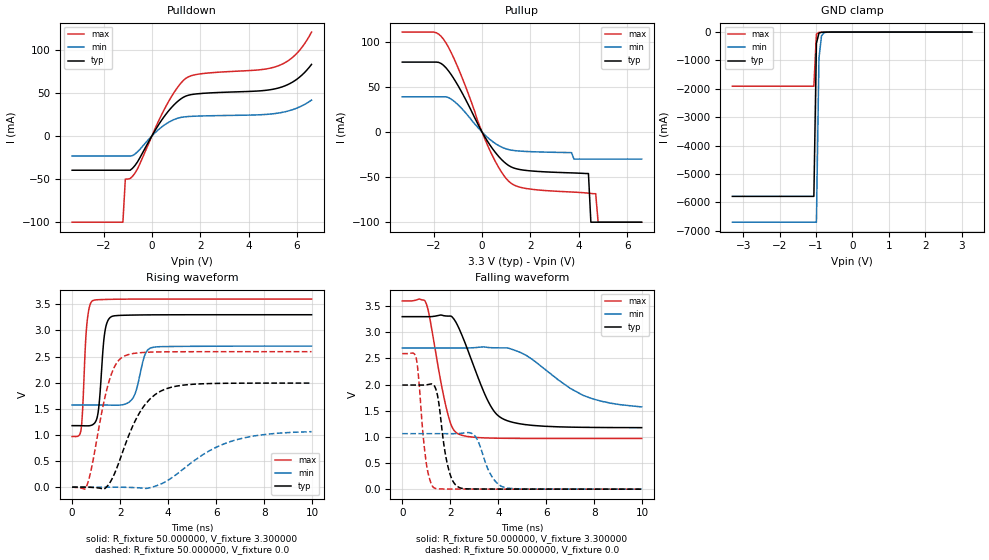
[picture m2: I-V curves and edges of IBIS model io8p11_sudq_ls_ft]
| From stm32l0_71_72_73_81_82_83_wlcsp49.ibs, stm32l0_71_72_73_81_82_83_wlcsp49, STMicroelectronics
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|   Model io8p11_sudq_ls_ft
[Model]  io8p11_sudq_ls_ft
Model_type I/O
Polarity   Non-Inverting
Enable   Active-Low
Vinl =   0.990000V
Vinh =   2.310000V
Vmeas =  1.650000V
Cref =   50.000000pF
Rref =   100.000000M
Vref =   0.0V
C_comp   2.343000pF   2.309800pF   2.393900pF
[Temperature Range]   25.000000   0.125000k   -40.000000
[Pullup Reference]   3.300000V   2.700000V   3.600000V
[Pulldown Reference]   0.0V   0.0V   0.0V
[POWER Clamp Reference]   3.300000V   2.700000V   3.600000V
[GND Clamp Reference]   0.0V   0.0V   0.0V
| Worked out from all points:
|   slope of the pulldown table from 0 to 0.495 V, typ, clamps not added: 22.6 ohm
|   slope of the pullup table from 0 to 0.495 V, typ, clamps not added: 23.9 ohm
|   GND clamp passes 1 mA (typ) near -0.64 V on its own axis
|   rising waveform, R_fixture 50.000000, V_fixture 3.300000: 20-80 % time 209ps typ, 360ps min, 167ps max; typ from 1.18 V to 3.3 V
|   rising waveform, R_fixture 50.000000, V_fixture 0.0: 20-80 % time 1.18ns typ, 2.2ns min, 697ps max; typ from 0 V to 1.99 V
|   falling waveform, R_fixture 50.000000, V_fixture 3.300000: 20-80 % time 1.12ns typ, 2.08ns min, 643ps max; typ from 3.3 V to 1.18 V
|   falling waveform, R_fixture 50.000000, V_fixture 0.0: 20-80 % time 383ps typ, 558ps min, 304ps max; typ from 1.99 V to 0 V
[Pulldown]
|Voltage   I(typ)   I(min)   I(max)
-3.3V     -39.8mA    -23.37mA   -100mA
-1.2V     -39.8mA    -23.37mA   -100mA
-1.1V     -39.8mA    -23.37mA   -50.1mA
-900mV    -39.8mA    -23.37mA   -49.43mA
-700mV    -34.25mA   -21mA      -43.13mA
600mV     25.84mA    14.18mA    35.34mA
1V        38.32mA    19.82mA    53.81mA
1.4V      46.09mA    22.19mA    66.63mA
2V        49.05mA    23.02mA    71.83mA
5.2V      55.23mA    26.32mA    80.92mA
6V        65.76mA    32.26mA    95.84mA
6.6V      82.81mA    41.43mA    120.2mA
[Pullup]
|Voltage   I(typ)   I(min)   I(max)
-3.3V     77.63mA    39.16mA    110.9mA
-2V       77.63mA    39.16mA    110.9mA
-1.6V     74.23mA    39.16mA    103.2mA
-900mV    47.13mA    27.82mA    65.37mA
300mV     -13.29mA   -7.65mA    -18.99mA
1.2V      -38.62mA   -20mA      -56.79mA
3.7V      -45.29mA   -22.8mA    -66.5mA
4.4V      -46mA      -30mA      -67.77mA
4.5V      -100mA     -30mA      -68.06mA
4.7V      -100mA     -30mA      -68.4mA
4.8V      -100mA     -30mA      -100mA
6.6V      -100mA     -30mA      -100mA
[GND_clamp]
|Voltage   I(typ)   I(min)   I(max)
-3.3V     -5.787A    -6.696A    -1.906A
-1.06V    -5.787A    -6.696A    -1.906A
-990mV    -393.4mA   -6.696A    -70.75mA
-920mV    -33.02mA   -919.4mA   -10.9mA
-850mV    -6.829mA   -131.3mA   -6.521mA
-780mV    -3.478mA   -21.06mA   -4.208mA
3.28V     0A         0A         0A
[POWER_clamp]
|Voltage   I(typ)   I(min)   I(max)
-3.28V    0A         0A         0A
0V        0A         0A         0A
[Ramp]
| variable   typ   min   max
dV/dt_r  1.19466/1.17578n   0.61164/2.08555n   1.55562/0.69590n
dV/dt_f  1.27212/1.11937n   0.59256/1.87709n   1.57784/0.64179n
R_load = 50.000000
[Rising Waveform]
R_fixture= 50.000000
V_fixture= 3.300000
V_fixture_min= 2.700000
V_fixture_max= 3.600000
|time   V(typ)   V(min)   V(max)
0s        1.177V     1.573V     969.2mV
380.4ps   1.176V     1.573V     1.129V
600.6ps   1.173V     1.573V     3.051V
860.9ps   1.196V     1.573V     3.57V
1.101ns   1.494V     1.573V     3.588V
1.381ns   3.02V      1.572V     3.592V
1.642ns   3.264V     1.569V     3.595V
2.523ns   3.294V     1.699V     3.599V
3.283ns   3.298V     2.666V     3.6V
9.97ns    3.3V       2.7V       3.6V
[Rising Waveform]
R_fixture= 50.000000
V_fixture= 0.0
V_fixture_min= 0.0
V_fixture_max= 0.0
|time   V(typ)   V(min)   V(max)
0s        -3.21uV    7.798uV    -231.3uV
620.6ps   -747.1uV   -8.107uV   39.58mV
820.8ps   -5.23mV    3.783uV    394.6mV
1.502ns   39.32mV    181.5uV    1.968V
1.802ns   299.1mV    -186.8uV   2.336V
2.122ns   696.8mV    -2.276mV   2.496V
3.003ns   1.56V      -23.84mV   2.579V
3.904ns   1.88V      106.7mV    2.59V
6.527ns   1.988V     862.3mV    2.593V
9.97ns    1.992V     1.062V     2.593V
[Falling Waveform]
R_fixture= 50.000000
V_fixture= 3.300000
V_fixture_min= 2.700000
V_fixture_max= 3.600000
|time   V(typ)   V(min)   V(max)
0s        3.3V       2.7V       3.6V
1.001ns   3.299V     2.7V       3.546V
1.842ns   3.312V     2.7V       1.541V
2.062ns   3.3V       2.7V       1.202V
2.302ns   3.134V     2.7V       1.065V
3.524ns   1.731V     2.714V     979.4mV
4.144ns   1.357V     2.702V     973.5mV
5.205ns   1.231V     2.547V     970.4mV
7.548ns   1.183V     1.791V     969.3mV
9.97ns    1.177V     1.573V     969.2mV
[Falling Waveform]
R_fixture= 50.000000
V_fixture= 0.0
V_fixture_min= 0.0
V_fixture_max= 0.0
|time   V(typ)   V(min)   V(max)
0s        1.992V     1.062V     2.593V
580.6ps   1.992V     1.062V     2.506V
981ps     1.994V     1.062V     567.6mV
1.341ns   1.973V     1.062V     20.38mV
1.902ns   434.4mV    1.062V     2.611mV
2.382ns   29.58mV    1.066V     1.674mV
3.043ns   3.182mV    1.008V     804.2uV
3.664ns   2.008mV    295mV      314.4uV
4.264ns   1.329mV    31.54mV    59.29uV
9.97ns    -3.21uV    7.798uV    -231.3uV
